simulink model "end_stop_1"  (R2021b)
settings: Solver=VariableStepAuto  StartTime=0.0  StopTime=20  RelTol=1e-3
libraries: fl_lib x9, nesl_utility x4

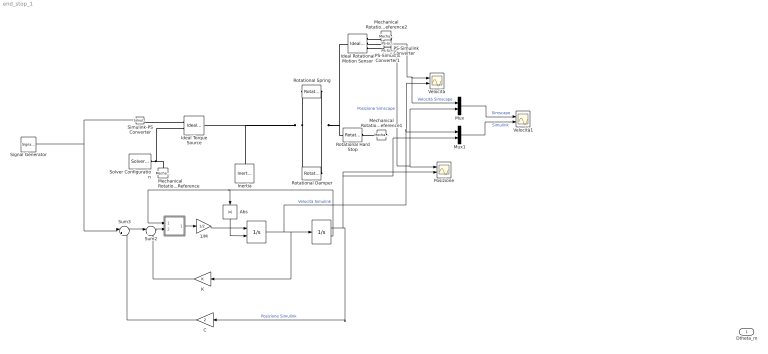
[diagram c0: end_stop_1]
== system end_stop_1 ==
  " " : Integrator  ExternalReset=rising
  "  " : Integrator  LimitOutput=on  UpperSaturationLimit=1  LowerSaturationLimit=-1  ShowSaturationPort=on
  "                       " : Subsystem
  1/M : Gain  Gain=1/2
  Abs : Abs
  C : Gain  Gain=2
  Ideal Rotational Motion Sensor : fl_lib/Mechanical/Mechanical Sensors/Ideal Rotational Motion Sensor  wrap_angle=simscape.enum.onoff.off  offset=0 rad
  Ideal Torque Source : fl_lib/Mechanical/Mechanical Sources/Ideal Torque Source
  Inertia : fl_lib/Mechanical/Rotational Elements/Inertia  inertia=2 kg*m^2  num_ports=foundation.enum.numPorts2.one  w_specify=off  w_priority=High  w=0 rad/s  w_nominal_specify=off  w_nominal_unit=rad/s  w_nominal_value=1  t_specify=off  t_priority=None  t=0 N*m  t_nominal_specify=off  t_nominal_unit=N*m  t_nominal_value=1
  K : Gain
  Mechanical Rotational Reference : fl_lib/Mechanical/Rotational Elements/Mechanical Rotational Reference
  Mechanical Rotational Reference1 : fl_lib/Mechanical/Rotational Elements/Mechanical Rotational Reference
  Mechanical Rotational Reference2 : fl_lib/Mechanical/Rotational Elements/Mechanical Rotational Reference
  Mux : Mux  Inputs=2
  Mux1 : Mux  Inputs=2
  PS-Simulink Converter : nesl_utility/PS-Simulink Converter  PhysicalDomain=network_engine_domain  SubClassName=ps_output  LeftPortType=input  RightPortType=output  PseudoPeriodic=off  Frequencies=[]  Unit=inherit  AffineConversion=off
  PS-Simulink Converter1 : nesl_utility/PS-Simulink Converter  PhysicalDomain=network_engine_domain  SubClassName=ps_output  LeftPortType=input  RightPortType=output  PseudoPeriodic=off  Frequencies=[]  Unit=inherit  AffineConversion=off
  Posizione : Scope  NumInputPorts=2
  Rotational Damper : fl_lib/Mechanical/Rotational Elements/Rotational Damper  D=2 N*m/(rad/s)  w_specify=off  w_priority=None  w=0 rad/s  w_nominal_specify=off  w_nominal_unit=rad/s  w_nominal_value=1  t_specify=off  t_priority=None  t=0 N*m  t_nominal_specify=off  t_nominal_unit=N*m  t_nominal_value=1
  Rotational Hard Stop : fl_lib/Mechanical/Rotational Elements/Rotational Hard Stop  upper_bnd=1 rad  lower_bnd=-1 rad  stiff_up=1e6 N*m/rad  stiff_low=1e6 N*m/rad  D_up=0.01 N*m/(rad/s)  D_low=0.01 N*m/(rad/s)  model=simscape.enum.hardstop.smooth  transition=0.001 rad  w_specify=off  w_priority=None  w=0 rad/s  w_nominal_specify=off  w_nominal_unit=rad/s  w_nominal_value=1  t_specify=off  t_priority=None  t=0 N*m  t_nominal_specify=off  t_nominal_unit=N*m  t_nominal_value=1  phi_specify=off  phi_priority=High  phi=0 rad  phi_nominal_specify=off  phi_nominal_unit=rad  phi_nominal_value=1
  Rotational Spring : fl_lib/Mechanical/Rotational Elements/Rotational Spring  spr_rate=1 N*m/rad  w_specify=off  w_priority=None  w=0 rad/s  w_nominal_specify=off  w_nominal_unit=rad/s  w_nominal_value=1  t_specify=off  t_priority=None  t=0 N*m  t_nominal_specify=off  t_nominal_unit=N*m  t_nominal_value=1  phi_specify=off  phi_priority=High  phi=0 rad  phi_nominal_specify=off  phi_nominal_unit=rad  phi_nominal_value=1
  Signal Generator : SignalGenerator  WaveForm=square  Amplitude=100  Frequency=2  Units=rad/sec
  Simulink-PS Converter : nesl_utility/Simulink-PS Converter  PhysicalDomain=network_engine_domain  SubClassName=ps_input  LeftPortType=input  RightPortType=output  PseudoPeriodic=off  Frequencies=[]  NoiseDistribution=none  NoiseParameters=[]  Unit=1  AffineConversion=off  FilteringAndDerivatives=provide  SimscapeFilterOrder=1  InputFilterTimeConstant=0.001  UdotUserProvided=0
  Solver Configuration : nesl_utility/Solver Configuration  PhysicalDomain=network_engine_domain  SubClassName=solver  LeftPortType=input  RightPortType=generic  Tones=[]  Harmonics=[]  SimulateNoise=off  Profile=off  UseLocalSampling=off  EnableSwitchedLinearOptims=on  FrequencyDomain=off  UseCCode=off  RelTol=0.001  AbsTol=1e-06  MinStep=1e-09  ToWorkspace=off  RevertToSquareIcSolve=off  NumHomotopyIterations=100  PhasorMode=off  PhasorModeNumHarmonics=1  DoDC=off  ResidualTolerance=1e-09  UseLocalSolver=off  LocalSolverChoice=NE_BACKWARD_EULER_ADVANCER  LocalSolverSampleTime=0.001  DoFixedCost=off  MaxNonlinIter=3  MaxModeIter=2  ComputeImpulses=off  ImpulseIterations=2  LinearAlgebra=auto  EquationFormulation=NE_TIME_EF  DelaysMemoryBudget=1024  AutomaticFiltering=on  FilteringTimeConstant=0.001  PartitionStorageMethod=AS_NEEDED  PartitionMemoryBudget=1024  PartitionMethod=ROBUST
  Sum2 : Sum  Inputs=|+-
  Sum3 : Sum  Inputs=|+-
  Velocità : Scope  NumInputPorts=2
  Velocità1 : Scope  NumInputPorts=2
  Dtheta_m : Outport
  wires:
  PS-Simulink Converter1/1 -> Mux/1, Velocità/1  "Velocità Simscape"
  PS-Simulink Converter/1 -> Mux/2, Posizione/1  "Posizione Simscape"
  "                       "/1(Act) -> 1/M/1
  " "/1 -> Velocità/2, Mux1/1, K/1, "  "/1  "Velocità Simulink"
  Sum3/1 -> Sum2/1
  Sum2/1 -> "                       "/2(Act ThC)
  C/1 -> Sum3/2
  Abs/1 -> " "/2
  "  "/2 -> "                       "/1(Sat Port), Abs/1
  1/M/1 -> " "/1
  "  "/1 -> Mux1/2, Posizione/2, C/1  "Posizione Simulink"
  K/1 -> Sum2/2
  Signal Generator/1 -> Sum3/1, Simulink-PS Converter/1
  Mux/1 -> Velocità1/1  "Simscape"
  Mux1/1 -> Velocità1/2  "Simulink"
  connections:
  Rotational Spring/LConn1 -- Inertia/LConn1 -- Ideal Torque Source/LConn1 -- Rotational Damper/LConn1
  Solver Configuration/RConn1 -- Ideal Torque Source/RConn2 -- Mechanical Rotational Reference/LConn1
  Rotational Damper/RConn1 -- Rotational Hard Stop/LConn1 -- Ideal Rotational Motion Sensor/LConn1 -- Rotational Spring/RConn1
  PS-Simulink Converter1/LConn1 -- Ideal Rotational Motion Sensor/RConn2
  Simulink-PS Converter/RConn1 -- Ideal Torque Source/RConn1
  PS-Simulink Converter/LConn1 -- Ideal Rotational Motion Sensor/RConn3
  Rotational Hard Stop/RConn1 -- Mechanical Rotational Reference1/LConn1
  Mechanical Rotational Reference2/LConn1 -- Ideal Rotational Motion Sensor/RConn1

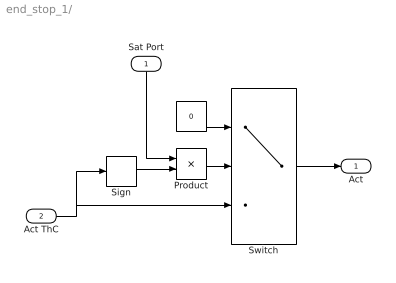
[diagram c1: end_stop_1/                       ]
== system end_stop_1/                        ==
  Sat Port : Inport
  Act ThC : Inport  Port=2
  "    " : Constant  Value=0
  Product : Product  RndMeth=Zero
  Sign : Signum
  Switch : Switch  Threshold=0.5
  Act : Outport
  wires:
  Act ThC/1 -> Switch/3, Sign/1
  Product/1 -> Switch/2
  Sign/1 -> Product/2
  "    "/1 -> Switch/1
  Switch/1 -> Act/1
  Sat Port/1 -> Product/1
